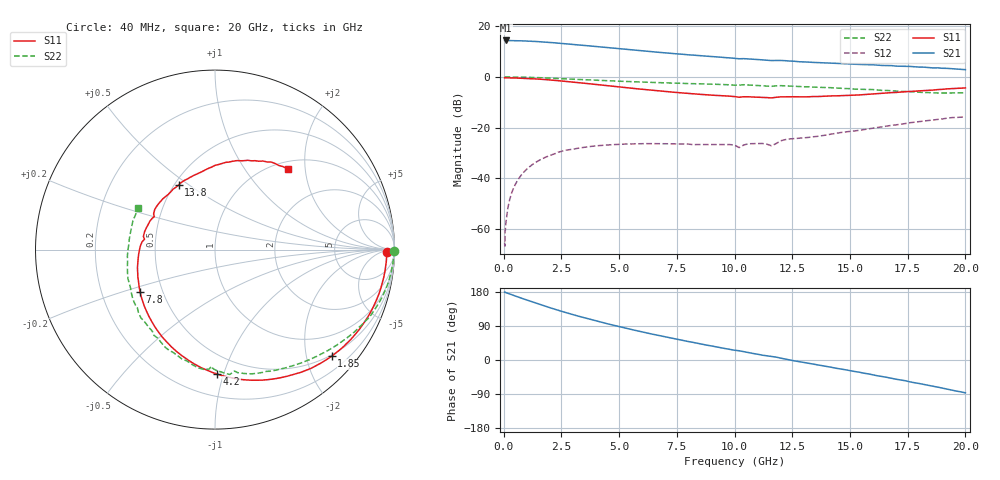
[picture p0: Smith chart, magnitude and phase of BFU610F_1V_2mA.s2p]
! Filename:  P:\Prog\Test\Noise\ATS_data\Testdata_Net\SplitFiles\BFU610_2W_A5_HighFreq_1V_2mA_D.s2p
! Date/Time: Wed 10/Aug/2011 16:54:35
! BFU610_2W_A5_HighFreq_1V_1mA_10mA_Bias2_R.s2p
! MDIF S-parameter v. bias file
! BFU610_2W_A5_HighFreq_1V_1mA_10mA
! Date/time Mon Aug 08 13:53:02 2011
! VAR V_out= 1.0002
! VAR I_out= 2.0000
! VAR V_in= 0.8730
! VAR I_in= 0.0155
! Device data file deembeded for feedlines and parallel
! Original file: \SplitFiles\BFU610_2W_A5_HighFreq_1V_2mA_R.s2p
! Feed-files: PR003V01_101208_Feed1.s2p, PR003V01_101208_Feed2.s2p
! Parallel-file: PR003V01_101208_Par.s2p
# MHz S MA R 50
!  Freq-MHz  S11-mag  S11-arg  S21-mag  S21-arg  S12-mag  S12-arg  S22-mag  S22-arg
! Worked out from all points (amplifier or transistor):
!   167 points, 40 MHz to 20 GHz, reference 50 ohm
!   highest |S21| = 14.3 dB at 80 MHz (marker M1)
!   |S21| within 3 dB of that: start of sweep to 4.711 GHz
!   unconditionally stable (mu >= 1): 6.511 GHz to end of sweep
!   at 550 MHz: K = 0.02, MSG = 27.9 dB, |S12| = -41.6 dB
!   at 4.2 GHz: K = 0.57, MSG = 19.4 dB, |S12| = -27.0 dB
!   at 20 GHz: K = 1.03, MAG = 8.2 dB, |S12| = -15.7 dB
!   S11 on the Smith chart (normalised r, x): 40 MHz: 40, -15; 1.85 GHz: 0.47, -2.50; 4.2 GHz: 0.36, -0.95; 7.8 GHz: 0.37, -0.23; 13.8 GHz: 0.53, +0.46; 20 GHz: 1.14, +1.62
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40  0.9571 -0.9  5.203 179.3  0.0005422 87.8  0.9952 -0.4
50  0.9535 -1.0  5.184 179.3  0.0004632 118.3  0.9951 -0.5
60  0.9594 -1.3  5.198 178.4  0.0008924 103.0  0.996 -0.6
80  0.957 -1.8  5.211 178.2  0.001121 91.4  0.996 -0.8
260  0.9555 -6.1  5.193 174.2  0.003834 89.3  0.9953 -2.9
600  0.9471 -14.1  5.166 166.8  0.009152 83.3  0.9905 -6.8
1300  0.9156 -30.2  5.005 152.0  0.01952 71.2  0.972 -14.4
1850  0.8807 -42.4  4.814 140.9  0.02661 62.6  0.9522 -20.1
2700  0.812 -60.3  4.487 125.0  0.03595 50.2  0.9123 -28.2
3400  0.7564 -74.2  4.19 113.0  0.0405 42.2  0.8826 -34.2
4200  0.6924 -89.2  3.883 100.1  0.04457 34.1  0.8499 -40.4
5400  0.607 -110.6  3.45 82.4  0.04768 24.8  0.8087 -49.3
6800  0.5245 -134.3  3.02 63.6  0.0483 17.1  0.7679 -59.0
7800  0.4788 -150.8  2.774 51.1  0.04774 14.1  0.7436 -65.7
9400  0.4264 -176.3  2.442 32.4  0.04645 13.8  0.7086 -76.9
10200  0.3969 171.6  2.271 24.4  0.04044 14.7  0.6856 -80.8
12000  0.4039 146.1  2.103 4.9  0.05504 30.7  0.6709 -95.1
13400  0.4099 124.7  1.927 -10.7  0.06605 24.8  0.6288 -108.8
13800  0.4128 119.4  1.889 -14.8  0.06949 25.1  0.6181 -112.4
16800  0.4895 83.1  1.665 -48.4  0.1109 13.4  0.534 -149.1
18400  0.5431 65.8  1.531 -67.2  0.1383 1.0  0.4898 -175.6
20000  0.6053 48.1  1.386 -86.7  0.1633 -15.2  0.4845 151.8
